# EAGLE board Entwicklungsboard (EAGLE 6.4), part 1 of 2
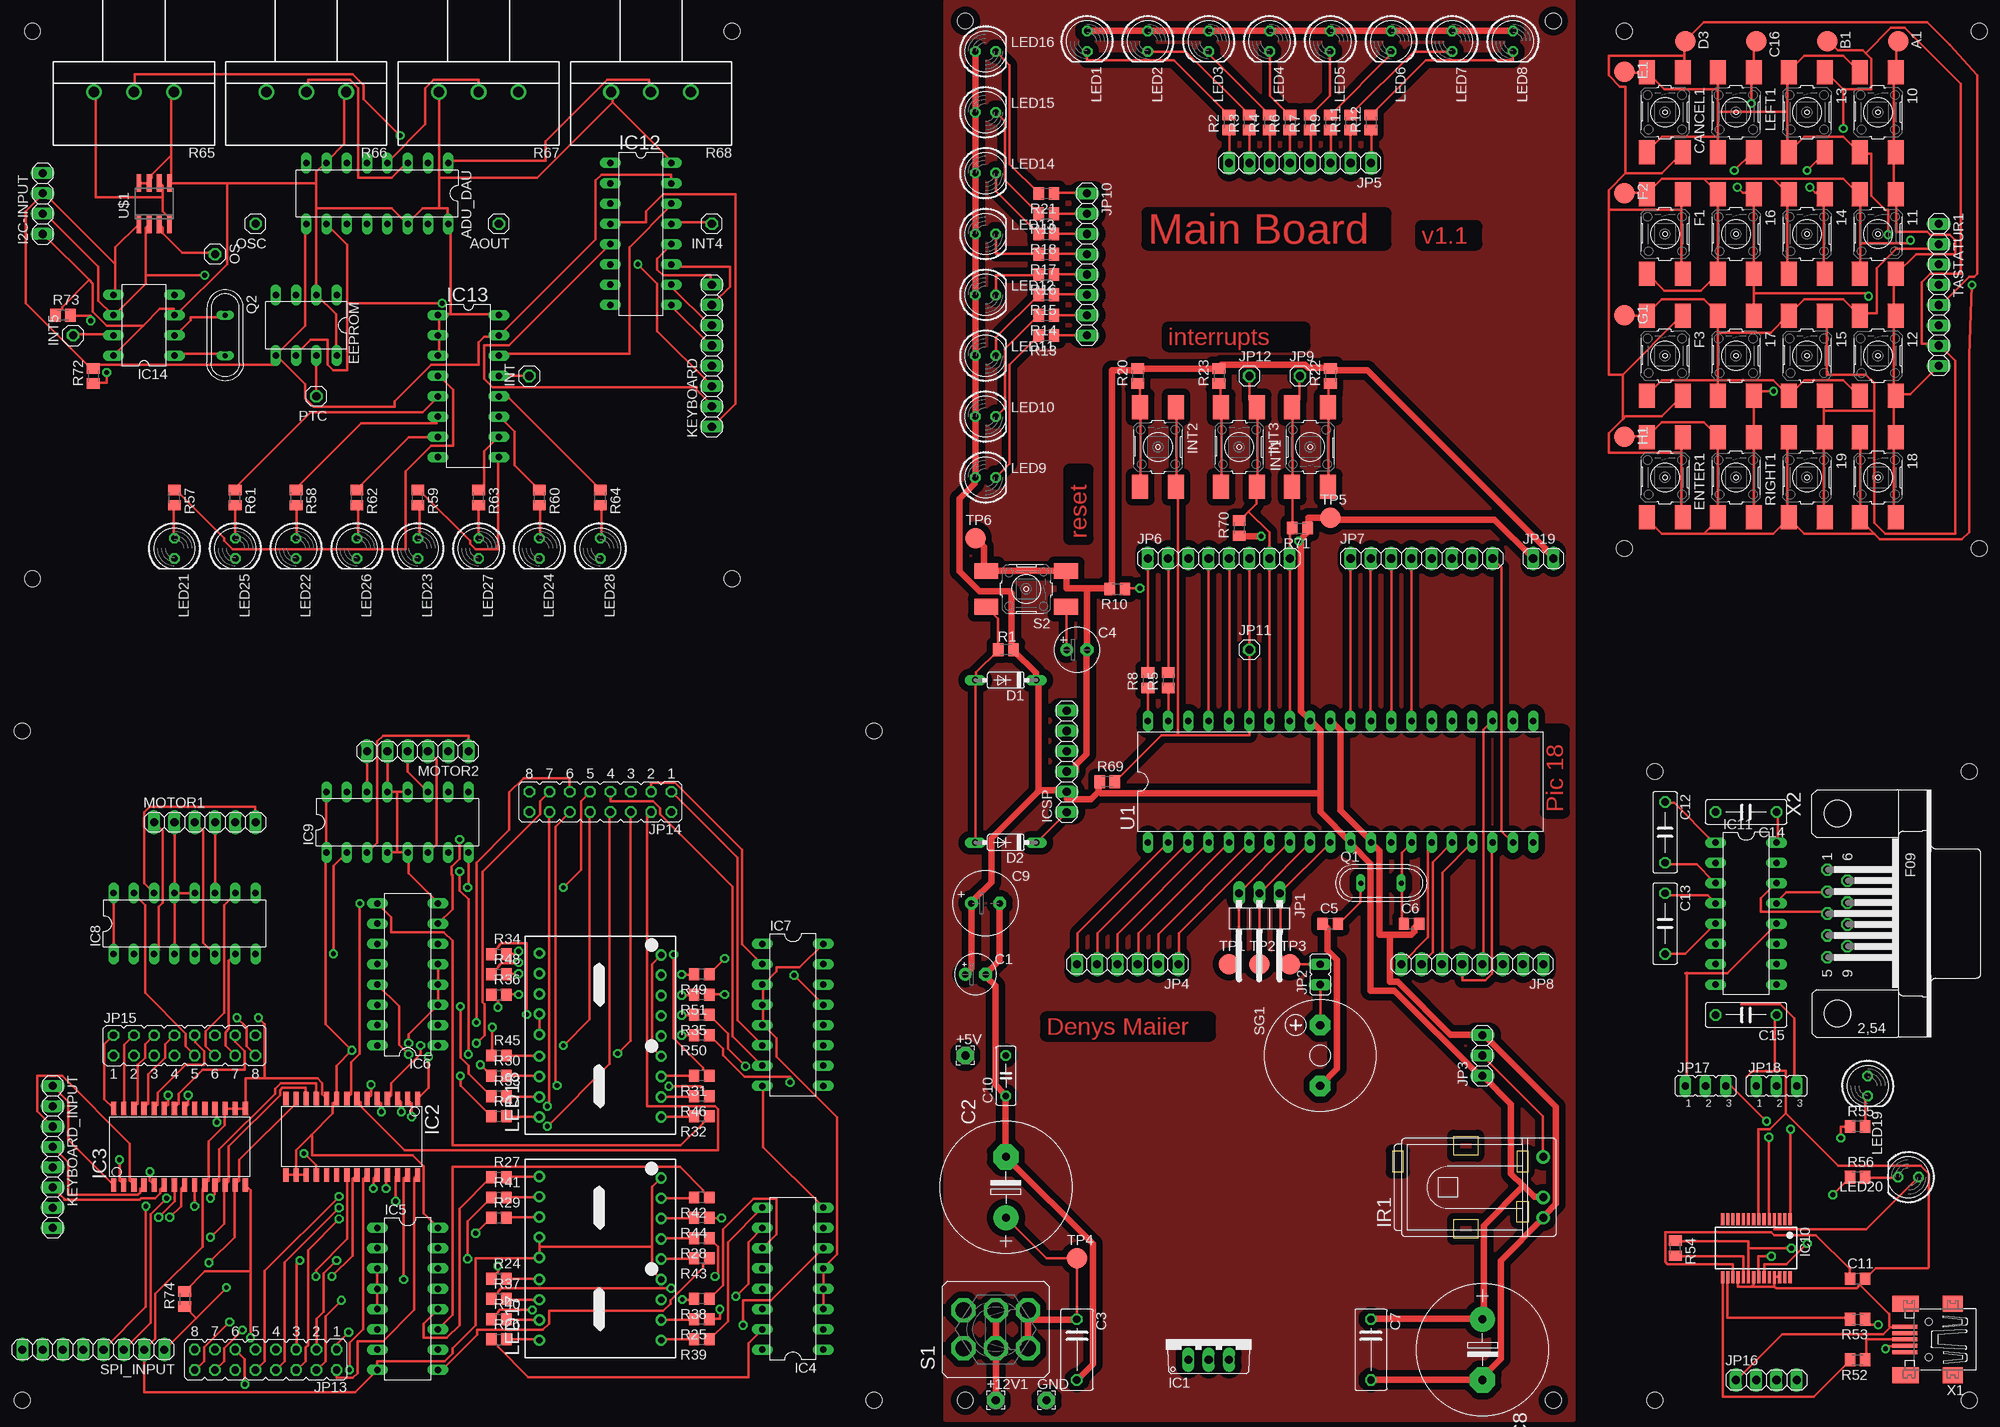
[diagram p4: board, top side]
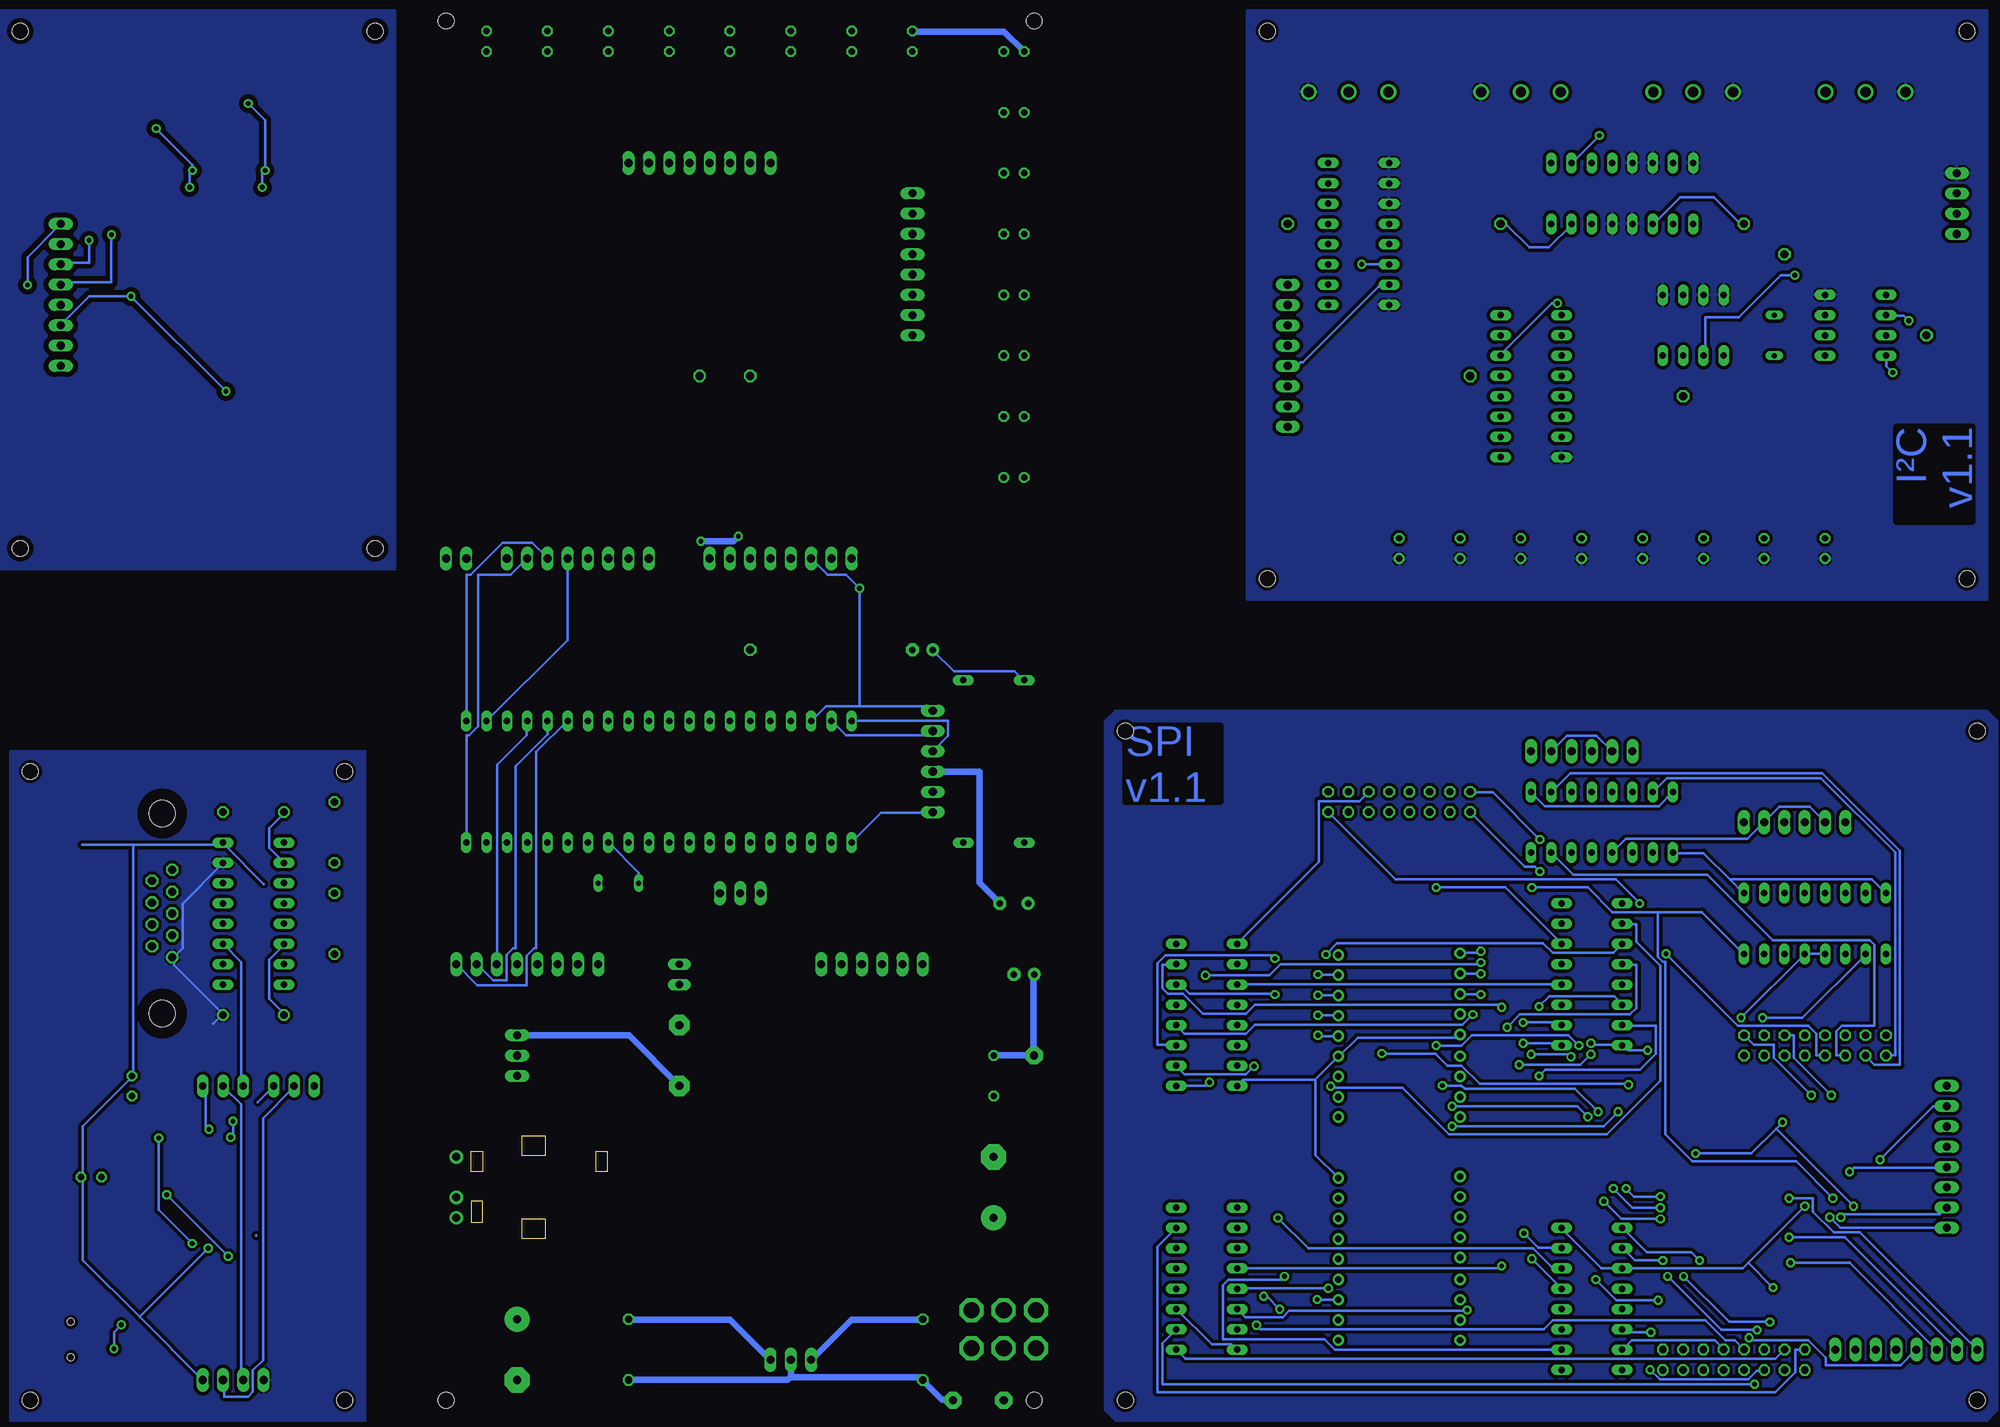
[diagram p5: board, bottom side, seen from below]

Size 17 x 12.8 mm. Coordinates in mm from the lower left corner, seen from the top.
Copper layers (1*16): Top 0.035mm / dielectric 1.5mm / Bottom 0.035mm
Design rules "default": minimum track width 0.25mm, minimum drill 0.6mm, track to track 0.25mm, track to pad 0.25mm, pad to pad 0.25mm, via to via 0.25mm, smd to smd 0.25mm, copper to edge 0.25mm, drill to drill 0.25mm, minimum pad ring 0.25mm, minimum via ring 0.25mm, stop-mask expansion 4mil, vias tented up to drill 0mil, thermal gap 0.25mm
Net classes: 0 default: width 0.3 mm; 1 GND: width 0.8 mm; 2 VCC: width 0.8 mm
Holes 2 mm at 73.51,86.41 73.51,151.18 29.06,151.18 29.06,86.41 -170.33,151.18 -82.7,151.18 -82.7,82.6 -170.33,82.6 -171.6,63.55 -64.92,63.55 -64.92,-20.27 -171.6,-20.27 -53.49,152.45 20.17,152.45 -53.49,-20.27 20.17,-20.27 72.24,58.47 72.24,-20.27 32.87,-20.27 32.87,58.47

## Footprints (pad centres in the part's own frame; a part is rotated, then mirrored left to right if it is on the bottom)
RAFI = smd 3 x 2: 1 -5,2.25; 2 5,2.25; 3 -5,-2.25; 4 5,-2.25
2,15/1,0 = drill 1.016 pad 2.159 octagon: 1 0,0
B2,54 = smd 2.54 x 2.54: TP 0,0
DIL16 = drill 0.813 long: 1 -8.89,-3.81; 2 -6.35,-3.81; 3 -3.81,-3.81; 4 -1.27,-3.81; 5 1.27,-3.81; 6 3.81,-3.81; 7 6.35,-3.81; 8 8.89,-3.81; 9 8.89,3.81; 10 6.35,3.81; 11 3.81,3.81; 12 1.27,3.81; 13 -1.27,3.81; 14 -3.81,3.81; 15 -6.35,3.81; 16 -8.89,3.81
1X01 = drill 1.016 octagon: 1 0,0
E2,5-5 = drill 0.813 pad 1.6: + -1.27,0 | drill 0.813 pad 1.6 octagon: - 1.27,0
E7,5-16 = drill 1.016 pad 3.15: + -3.81,0 | drill 1.016 pad 3.15 octagon: - 3.81,0
C075-042X103 = drill 0.914 octagon: 1 -3.81,0; 2 3.81,0
E2,5-6 = drill 0.813 pad 1.6: + -1.27,0 | drill 0.813 pad 1.6 octagon: - 1.27,0
C0805 = smd 1.3 x 1.5: 1 -0.95,0; 2 0.95,0
E3,5-8 = drill 0.813 pad 1.6: + -1.778,0 | drill 0.813 pad 1.6 octagon: - 1.778,0
C050-025X075 = drill 0.813 octagon: 1 -2.54,0; 2 2.54,0
C075-032X103 = drill 0.914 octagon: 1 -3.81,0; 2 3.81,0
DO35-7 = drill 0.813 long: A 3.81,0; C -3.81,0
DIL08 = drill 0.813 long: 1 -3.81,-3.81; 2 -1.27,-3.81; 3 1.27,-3.81; 4 3.81,-3.81; 5 3.81,3.81; 6 1.27,3.81; 7 -1.27,3.81; 8 -3.81,3.81
1X04 = drill 1.016 long: 1 -3.81,0; 2 -1.27,0; 3 1.27,0; 4 3.81,0
TO220V = drill 1.016 long: 1 -2.54,-2.54; 2 0,-2.54; 3 2.54,-2.54
SO28W = smd 0.65 x 1.7: 1 -7.62,-4.78; 2 -6.35,-4.78; 3 -5.08,-4.78; 4 -3.81,-4.78; 5 -2.54,-4.78; 6 -1.27,-4.78; 7 0,-4.78; 8 1.27,-4.78; 9 2.54,-4.78; 10 3.81,-4.78; 11 5.08,-4.78; 12 6.35,-4.78; 13 7.62,-4.78; 14 8.89,-4.78; 15 8.89,4.78; 16 7.62,4.78; 17 6.35,4.78; 18 5.08,4.78; 19 3.81,4.78; 20 2.54,4.78; 21 1.27,4.78; 22 0,4.78; 23 -1.27,4.78; 24 -2.54,4.78; 25 -3.81,4.78; 26 -5.08,4.78; 27 -6.35,4.78; 28 -7.62,4.78
SSOP28 = smd 0.4 x 1.5: 1 -4.225,-3.625; 2 -3.575,-3.625; 3 -2.925,-3.625; 4 -2.275,-3.625; 5 -1.625,-3.625; 6 -0.975,-3.625; 7 -0.325,-3.625; 8 0.325,-3.625; 9 0.975,-3.625; 10 1.625,-3.625; 11 2.275,-3.625; 12 2.925,-3.625; 13 3.575,-3.625; 14 4.225,-3.625; 15 4.225,3.625; 16 3.575,3.625; 17 2.925,3.625; 18 2.275,3.625; 19 1.625,3.625; 20 0.975,3.625; 21 0.325,3.625; 22 -0.325,3.625; 23 -0.975,3.625; 24 -1.625,3.625; 25 -2.275,3.625; 26 -2.925,3.625; 27 -3.575,3.625; 28 -4.225,3.625
1X06 = drill 1.016 long: 1 -6.35,0; 2 -3.81,0; 3 -1.27,0; 4 1.27,0; 5 3.81,0; 6 6.35,0
TSOP17_TB1 = drill 1 pad 1.676: GND 0,-3.81; VO 0,3.81; VS 0,-1.27
1X03/90 = drill 1.016 long: 1 -2.54,-3.81; 2 0,-3.81; 3 2.54,-3.81
JP1 = drill 0.914 long: 1 0,-1.27; 2 0,1.27
1X03 = drill 1.016 long: 1 -2.54,0; 2 0,0; 3 2.54,0
1X08 = drill 1.016 long: 1 -8.89,0; 2 -6.35,0; 3 -3.81,0; 4 -1.27,0; 5 1.27,0; 6 3.81,0; 7 6.35,0; 8 8.89,0
JP8Q = drill 0.914 octagon: 1 -8.89,-1.27; 2 -8.89,1.27; 3 -6.35,-1.27; 4 -6.35,1.27; 5 -3.81,-1.27; 6 -3.81,1.27; 7 -1.27,-1.27; 8 -1.27,1.27; 9 1.27,-1.27; 10 1.27,1.27; 11 3.81,-1.27; 12 3.81,1.27; 13 6.35,-1.27; 14 6.35,1.27; 15 8.89,-1.27; 16 8.89,1.27
JP2 = drill 0.914 long: 1 -2.54,0; 2 0,0; 3 2.54,0
1X02 = drill 1.016 long: 1 -1.27,0; 2 1.27,0
LED5MM = drill 0.813 octagon: A -1.27,0; K 1.27,0
DA56 = drill 0.8 pad 1.422: 1 -10.26,-7.62; 2 -7.72,-7.62; 3 -5.18,-7.62; 4 -2.64,-7.62; 5 -0.1,-7.62; 6 2.44,-7.62; 7 4.98,-7.62; 8 7.52,-7.62; 9 10.06,-7.62; 10 10.26,7.62; 11 7.72,7.62; 12 5.18,7.62; 13 2.64,7.62; 14 0.1,7.62; 15 -2.64,7.62; 16 -5.18,7.62; 17 -7.72,7.62; 18 -10.26,7.62
QS = drill 0.61 long: 1 -2.54,0; 2 2.54,0
M0805 = smd 1.3 x 1.6: 1 -0.95,0; 2 0.95,0
R0805 = smd 1.3 x 1.5: 1 -0.95,0; 2 0.95,0
CIP20C-6MM = drill 1.3 pad 1.93: A -5,0; E 5,0; S 0,0
320-938 = drill 2.007 octagon: 1 -2.388,4.013; 2 -2.388,0; 3 -2.388,-4.013; 4 2.388,4.013; 5 2.388,0; 6 2.388,-4.013
F/CM12P = drill 1.016 pad 2.54 octagon: + 3.81,0; - -3.81,0
DIL40 = drill 0.813 long: 1 -24.13,-7.62; 2 -21.59,-7.62; 3 -19.05,-7.62; 4 -16.51,-7.62; 5 -13.97,-7.62; 6 -11.43,-7.62; 7 -8.89,-7.62; 8 -6.35,-7.62; 9 -3.81,-7.62; 10 -1.27,-7.62; 11 1.27,-7.62; 12 3.81,-7.62; 13 6.35,-7.62; 14 8.89,-7.62; 15 11.43,-7.62; 16 13.97,-7.62; 17 16.51,-7.62; 18 19.05,-7.62; 19 21.59,-7.62; 20 24.13,-7.62; 21 24.13,7.62; 22 21.59,7.62; 23 19.05,7.62; 24 16.51,7.62; 25 13.97,7.62; 26 11.43,7.62; 27 8.89,7.62; 28 6.35,7.62; 29 3.81,7.62; 30 1.27,7.62; 31 -1.27,7.62; 32 -3.81,7.62; 33 -6.35,7.62; 34 -8.89,7.62; 35 -11.43,7.62; 36 -13.97,7.62; 37 -16.51,7.62; 38 -19.05,7.62; 39 -21.59,7.62; 40 -24.13,7.62
SO08 = smd 0.6 x 2.2: 1 -1.905,-2.6; 2 -0.635,-2.6; 3 0.635,-2.6; 4 1.905,-2.6; 5 1.905,2.6; 6 0.635,2.6; 7 -0.635,2.6; 8 -1.905,2.6
32005-301 = smd 3.1 x 0.5: 1 3,1.6; 2 3,0.8; 3 3,0; 4 3,-0.8; 5 3,-1.6 | smd 2.5 x 2: M1 -3,-4.45; M2 -3,4.45 | smd 3.3 x 2: M3 2.9,4.45; M4 2.9,-4.45 | hole 0.9: 0,2.2; 0,-2.2
F09H = drill 1.016 octagon: 1 -5.486,-1.27; 2 -2.743,-1.27; 3 0,-1.27; 4 2.743,-1.27; 5 5.486,-1.27; 6 -4.115,1.27; 7 -1.372,1.27; 8 1.372,1.27; 9 4.115,1.27 | hole 3.302: -12.522,0; 12.522,0

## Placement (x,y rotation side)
10  [RAFI]  60.81,141.02 270 top  (outside the outline)
11  [RAFI]  60.81,125.78 270 top  (outside the outline)
12  [RAFI]  60.81,110.54 270 top  (outside the outline)
13  [RAFI]  51.92,141.02 270 top  (outside the outline)
14  [RAFI]  51.92,125.78 270 top  (outside the outline)
15  [RAFI]  51.92,110.54 270 top  (outside the outline)
16  [RAFI]  43.03,125.78 270 top  (outside the outline)
17  [RAFI]  43.03,110.54 270 top  (outside the outline)
18  [RAFI]  60.81,95.3 270 top  (outside the outline)
19  [RAFI]  51.92,95.3 270 top  (outside the outline)
+5V  [2,15/1,0]  -53.49,22.91 0 top  (outside the outline)
+12V1  [2,15/1,0]  -49.68,-20.27 0 top  (outside the outline)
A1  TPB2,54  [B2,54]  63.35,149.91 270 top  (outside the outline)
ADU_DAU  PCF8591P  [DIL16]  -127.15,130.86 180 top  (outside the outline)
AOUT  [1X01]  -111.91,127.05 180 top  (outside the outline)
B1  TPB2,54  [B2,54]  54.46,149.91 270 top  (outside the outline)
C1  [E2,5-5]  -52.22,33.07 0 top  (outside the outline)
C2  470uF  [E7,5-16]  -48.41,6.4 90 top  (outside the outline)
C3  0,1uF  [C075-042X103]  -39.52,-13.92 270 top  (outside the outline)
C4  10uF  [E2,5-6]  -39.52,73.71 0 top  (outside the outline)
C5  [C0805]  -7.77,39.42 0 top  (outside the outline)
C6  [C0805]  2.39,39.42 0 top  (outside the outline)
C7  0,1uF  [C075-042X103]  -2.69,-13.92 270 top  (outside the outline)
C8  470uF  [E7,5-16]  11.28,-13.92 270 top  (outside the outline)
C9  [E3,5-8]  -50.95,41.96 0 top  (outside the outline)
C10  [C050-025X075]  -48.41,20.37 90 top  (outside the outline)
C11  [C0805]  58.27,-5.03 0 top  (outside the outline)
C12  100nF  [C075-032X103]  34.14,50.85 270 top  (outside the outline)
C13  100nF  [C075-032X103]  34.14,39.42 270 top  (outside the outline)
C14  100nF  [C075-032X103]  44.3,53.39 180 top  (outside the outline)
C15  100nF  [C075-032X103]  44.3,27.99 180 top  (outside the outline)
C16  TPB2,54  [B2,54]  45.57,149.91 270 top  (outside the outline)
CANCEL1  [RAFI]  34.14,141.02 270 top  (outside the outline)
D1  1N4148DO35-7  [DO35-7]  -48.41,69.9 180 top  (outside the outline)
D2  1N4148DO35-7  [DO35-7]  -48.41,49.58 180 top  (outside the outline)
D3  TPB2,54  [B2,54]  36.68,149.91 270 top  (outside the outline)
E1  TPB2,54  [B2,54]  29.06,146.1 270 top  (outside the outline)
EEPROM  PCF8582C-2P/03  [DIL08]  -136.04,114.35 180 top  (outside the outline)
ENTER1  [RAFI]  34.14,95.3 270 top  (outside the outline)
F1  [RAFI]  34.14,125.78 270 top  (outside the outline)
F2  TPB2,54  [B2,54]  29.06,130.86 270 top  (outside the outline)
F3  [RAFI]  34.14,110.54 270 top  (outside the outline)
G1  TPB2,54  [B2,54]  29.06,115.62 270 top  (outside the outline)
GND  [2,15/1,0]  -43.33,-20.27 0 top  (outside the outline)
H1  TPB2,54  [B2,54]  29.06,100.38 270 top  (outside the outline)
I2C-INPUT  [1X04]  -169.06,129.59 90 top  (outside the outline)
IC1  7805TV  [TO220V]  -23.01,-12.65 0 top  (outside the outline)
IC2  MCP23S17SO  [SO28W]  -129.69,12.75 180 top  (outside the outline)
IC3  MCP23S17SO  [SO28W]  -152.55,11.48 0 top  (outside the outline)
IC4  74LS48N  [DIL16]  -75.08,-5.03 90 top  (outside the outline)
IC5  74LS48N  [DIL16]  -123.34,-7.57 270 top  (outside the outline)
IC6  74LS48N  [DIL16]  -123.34,33.07 90 top  (outside the outline)
IC7  74LS48N  [DIL16]  -75.08,27.99 270 top  (outside the outline)
IC8  L293D  [DIL16]  -151.28,39.42 0 top  (outside the outline)
IC9  L293D  [DIL16]  -124.61,52.12 0 top  (outside the outline)
IC10  FT232RL  [SSOP28]  45.57,-1.22 180 top  (outside the outline)
IC11  MAX232  [DIL16]  44.3,40.69 270 top  (outside the outline)
IC12  PCF8574P  [DIL16]  -94.13,125.78 270 top  (outside the outline)
IC13  PCF8574P  [DIL16]  -115.72,106.73 270 top  (outside the outline)
IC14  PFC8583P  [DIL08]  -156.36,114.35 90 top  (outside the outline)
ICSP  [1X06]  -40.79,59.74 90 top  (outside the outline)
INT  [1X01]  -108.1,108 90 top  (outside the outline)
INT1  [RAFI]  -10.31,99.11 90 top  (outside the outline)
INT2  [RAFI]  -29.36,99.11 270 top  (outside the outline)
INT3  [RAFI]  -19.2,99.11 270 top  (outside the outline)
INT4  [1X01]  -85.24,127.05 180 top  (outside the outline)
INT5  [1X01]  -165.25,113.08 90 top  (outside the outline)
IR1  TSOP1736TB1  [TSOP17_TB1]  18.9,6.4 0 top
JP1  [1X03/90]  -16.66,39.42 180 top  (outside the outline)
JP2  [JP1]  -9.04,33.07 0 top  (outside the outline)
JP3  [1X03]  11.28,22.91 90 top  (outside the outline)
JP4  [1X06]  -33.17,34.34 180 top  (outside the outline)
JP5  [1X08]  -11.58,134.67 180 top  (outside the outline)
JP6  [1X08]  -21.74,85.14 0 top  (outside the outline)
JP7  [1X08]  3.66,85.14 0 top  (outside the outline)
JP8  [1X08]  10.01,34.34 180 top  (outside the outline)
JP9  [1X01]  -11.58,108 0 top  (outside the outline)
JP10  [1X08]  -38.25,121.97 270 top  (outside the outline)
JP11  [1X01]  -17.93,73.71 0 top  (outside the outline)
JP12  [1X01]  -17.93,108 0 top  (outside the outline)
JP13  [JP8Q]  -141.12,-15.19 180 top  (outside the outline)
JP14  [JP8Q]  -99.21,54.66 180 top  (outside the outline)
JP15  [JP8Q]  -151.28,24.18 0 top  (outside the outline)
JP16  [1X04]  46.84,-17.73 0 top  (outside the outline)
JP17  [JP2]  39.22,19.1 0 top  (outside the outline)
JP18  [JP2]  48.11,19.1 0 top  (outside the outline)
JP19  [1X02]  18.9,85.14 0 top  (outside the outline)
KEYBOARD  [1X08]  -85.24,110.54 90 top  (outside the outline)
KEYBOARD_INPUT  [1X08]  -167.79,10.21 270 top  (outside the outline)
LED1  [LED5MM]  -38.25,149.91 270 top  (outside the outline)
LED2  [LED5MM]  -30.63,149.91 270 top  (outside the outline)
LED3  [LED5MM]  -23.01,149.91 270 top  (outside the outline)
LED4  [LED5MM]  -15.39,149.91 270 top  (outside the outline)
LED5  [LED5MM]  -7.77,149.91 270 top  (outside the outline)
LED6  [LED5MM]  -0.15,149.91 270 top  (outside the outline)
LED7  [LED5MM]  7.47,149.91 270 top  (outside the outline)
LED8  [LED5MM]  15.09,149.91 270 top  (outside the outline)
LED9  [LED5MM]  -50.95,95.3 0 top  (outside the outline)
LED10  [LED5MM]  -50.95,102.92 0 top  (outside the outline)
LED11  [LED5MM]  -50.95,110.54 0 top  (outside the outline)
LED12  [LED5MM]  -50.95,118.16 0 top  (outside the outline)
LED13  [LED5MM]  -50.95,125.78 0 top  (outside the outline)
LED14  [LED5MM]  -50.95,133.4 0 top  (outside the outline)
LED15  [LED5MM]  -50.95,141.02 0 top  (outside the outline)
LED16  [LED5MM]  -50.95,148.64 0 top  (outside the outline)
LED17  DC56-11GWA  [DA56]  -99.21,-2.49 90 top  (outside the outline)
LED18  DC56-11GWA  [DA56]  -99.21,25.45 90 top  (outside the outline)
LED19  [LED5MM]  59.54,19.1 270 top  (outside the outline)
LED20  [LED5MM]  64.62,7.67 180 top  (outside the outline)
LED21  [LED5MM]  -152.55,86.41 270 top  (outside the outline)
LED22  [LED5MM]  -137.31,86.41 270 top  (outside the outline)
LED23  [LED5MM]  -122.07,86.41 270 top  (outside the outline)
LED24  [LED5MM]  -106.83,86.41 270 top  (outside the outline)
LED25  [LED5MM]  -144.93,86.41 270 top  (outside the outline)
LED26  [LED5MM]  -129.69,86.41 270 top  (outside the outline)
LED27  [LED5MM]  -114.45,86.41 270 top  (outside the outline)
LED28  [LED5MM]  -99.21,86.41 270 top  (outside the outline)
LEFT1  [RAFI]  43.03,141.02 270 top  (outside the outline)
MOTOR1  [1X06]  -148.74,52.12 0 top  (outside the outline)
MOTOR2  [1X06]  -122.07,61.01 180 top  (outside the outline)
OS  [1X01]  -147.47,123.24 270 top  (outside the outline)
OSC  [1X01]  -142.39,127.05 180 top  (outside the outline)
PTC  [1X01]  -134.77,105.46 180 top  (outside the outline)
Q1  20Mhz  [QS]  -1.42,44.5 0 top  (outside the outline)
Q2  32.768kHz  [QS]  -146.2,113.08 270 top  (outside the outline)
R1  10k  [M0805]  -48.41,73.71 0 top  (outside the outline)
R2  330  [M0805]  -20.47,139.75 90 top  (outside the outline)
R3  [M0805]  -17.93,139.75 90 top  (outside the outline)
R4  [M0805]  -15.39,139.75 90 top  (outside the outline)
R5  10k  [M0805]  -28.09,69.9 90 top  (outside the outline)
R6  [M0805]  -12.85,139.75 90 top  (outside the outline)
R7  [M0805]  -10.31,139.75 90 top  (outside the outline)
R8  10k  [M0805]  -30.63,69.9 90 top  (outside the outline)
R9  [M0805]  -7.77,139.75 90 top  (outside the outline)
R10  10k  [M0805]  -34.44,81.33 180 top  (outside the outline)
R11  [M0805]  -5.23,139.75 90 top  (outside the outline)
R12  330  [M0805]  -2.69,139.75 90 top  (outside the outline)
R13  330  [M0805]  -43.33,113.08 180 top  (outside the outline)
R14  [M0805]  -43.33,115.62 180 top  (outside the outline)
R15  [M0805]  -43.33,118.16 180 top  (outside the outline)
R16  [M0805]  -43.33,120.7 180 top  (outside the outline)
R17  [M0805]  -43.33,123.24 180 top  (outside the outline)
R18  [M0805]  -43.33,125.78 180 top  (outside the outline)
R19  [M0805]  -43.33,128.32 180 top  (outside the outline)
R20  270  [M0805]  -31.9,108 90 top  (outside the outline)
R21  330  [M0805]  -43.33,130.86 180 top  (outside the outline)
R22  270  [M0805]  -7.77,108 90 top  (outside the outline)
R23  270  [M0805]  -21.74,108 90 top  (outside the outline)
R24  300  [R0805]  -111.91,-5.03 0 top  (outside the outline)
R25  300  [R0805]  -86.51,-10.11 180 top  (outside the outline)
R26  300  [R0805]  -111.91,-12.65 0 top  (outside the outline)
R27  300  [R0805]  -111.91,7.67 0 top  (outside the outline)
R28  300  [R0805]  -86.51,0.05 180 top  (outside the outline)
R29  300  [R0805]  -111.91,2.59 0 top  (outside the outline)
R30  300  [R0805]  -111.91,20.37 0 top  (outside the outline)
R31  300  [R0805]  -86.51,20.37 180 top  (outside the outline)
R32  300  [R0805]  -86.51,15.29 180 top  (outside the outline)
R33  300  [R0805]  -111.91,17.83 0 top  (outside the outline)
R34  300  [R0805]  -111.91,35.61 0 top  (outside the outline)
R35  300  [R0805]  -86.51,27.99 180 top  (outside the outline)
R36  300  [R0805]  -111.91,30.53 0 top  (outside the outline)
R37  300  [R0805]  -111.91,-7.57 0 top  (outside the outline)
R38  300  [R0805]  -86.51,-7.57 180 top  (outside the outline)
R39  300  [R0805]  -86.51,-12.65 180 top  (outside the outline)
R40  300  [R0805]  -111.91,-10.11 0 top  (outside the outline)
R41  300  [R0805]  -111.91,5.13 0 top  (outside the outline)
R42  300  [R0805]  -86.51,5.13 180 top  (outside the outline)
R43  300  [R0805]  -86.51,-2.49 180 top  (outside the outline)
R44  300  [R0805]  -86.51,2.59 180 top  (outside the outline)
R45  300  [R0805]  -111.91,22.91 0 top  (outside the outline)
R46  300  [R0805]  -86.51,17.83 180 top  (outside the outline)
R47  300  [R0805]  -111.91,15.29 0 top  (outside the outline)
R48  300  [R0805]  -111.91,33.07 0 top  (outside the outline)
R49  300  [R0805]  -86.51,33.07 180 top  (outside the outline)
R50  300  [R0805]  -86.51,25.45 180 top  (outside the outline)
R51  300  [R0805]  -86.51,30.53 180 top  (outside the outline)
R52  27R  [M0805]  58.27,-15.19 180 top  (outside the outline)
R53  27R  [M0805]  58.27,-10.11 180 top  (outside the outline)
R54  [M0805]  35.44,-1.22 270 top  (outside the outline)
R55  330  [M0805]  58.27,14.02 0 top  (outside the outline)
R56  330  [M0805]  58.27,7.67 0 top  (outside the outline)
R57  330  [M0805]  -152.55,92.76 270 top  (outside the outline)
R58  330  [M0805]  -137.31,92.76 270 top  (outside the outline)
R59  330  [M0805]  -122.07,92.76 270 top  (outside the outline)
R60  330  [M0805]  -106.83,92.76 270 top  (outside the outline)
R61  330  [M0805]  -144.93,92.76 270 top  (outside the outline)
R62  330  [M0805]  -129.69,92.76 270 top  (outside the outline)
R63  330  [M0805]  -114.45,92.76 270 top  (outside the outline)
R64  330  [M0805]  -99.21,92.76 270 top  (outside the outline)
R65  [CIP20C-6MM]  -157.63,143.56 180 top  (outside the outline)
R66  [CIP20C-6MM]  -136.04,143.56 180 top  (outside the outline)
R67  [CIP20C-6MM]  -114.45,143.56 180 top  (outside the outline)
R68  [CIP20C-6MM]  -92.86,143.56 180 top  (outside the outline)
R69  4.7k  [M0805]  -35.71,57.2 0 top  (outside the outline)
R70  4.7k  [M0805]  -19.2,88.95 90 top  (outside the outline)
R71  4.7k  [M0805]  -11.58,88.95 180 top  (outside the outline)
R72  4.7k  [M0805]  -162.71,108 90 top  (outside the outline)
R73  4.7k  [M0805]  -166.52,115.62 0 top  (outside the outline)
R74  [M0805]  -151.28,-7.57 90 top  (outside the outline)
RIGHT1  [RAFI]  43.03,95.3 270 top  (outside the outline)
S1  [320-938]  -49.68,-11.38 90 top  (outside the outline)
S2  [RAFI]  -45.87,81.33 180 top  (outside the outline)
SG1  F/CM12P  [F/CM12P]  -9.04,22.91 90 top  (outside the outline)
SPI_INPUT  [1X08]  -162.71,-13.92 180 top  (outside the outline)
TASTATUR1  [1X08]  68.43,118.16 270 top  (outside the outline)
TP1  TPB2,54  [B2,54]  -20.47,34.34 0 top  (outside the outline)
TP2  TPB2,54  [B2,54]  -16.66,34.34 0 top  (outside the outline)
TP3  TPB2,54  [B2,54]  -12.85,34.34 0 top  (outside the outline)
TP4  TPB2,54  [B2,54]  -39.52,-2.49 0 top  (outside the outline)
TP5  TPB2,54  [B2,54]  -7.77,90.22 0 top  (outside the outline)
TP6  TPB2,54  [B2,54]  -52.22,87.68 0 top  (outside the outline)
U1  PIC18F4520-I/P  [DIL40]  -6.5,57.2 0 top  (outside the outline)
U$1  LM75AD  [SO08]  -155.09,129.59 0 top  (outside the outline)
U$2  [DINA4_L]  not placed on the board
X1  MINI-USB-32005-301  [32005-301]  67.16,-12.65 180 top  (outside the outline)
X2  [F09H]  55.73,40.69 270 top  (outside the outline)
